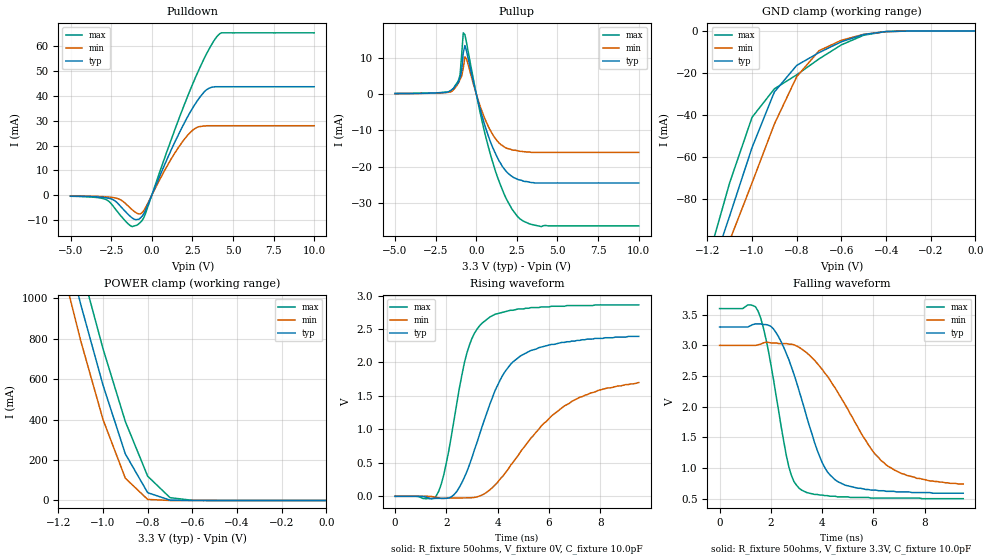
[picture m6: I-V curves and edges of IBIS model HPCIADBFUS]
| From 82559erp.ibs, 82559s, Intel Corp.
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[Model]   HPCIADBFUS
Model_type   I/O
Vinl  =   1.08V   | note : 0.3 * VCCmax
Vinh  =   1.5V   | note : 0.5 * VCCmin
|   typ   min  max
C_comp   2.7pF NA   NA
| note : on die power/gnd supply distribution R/L/C
|   are not included in the simulation
| note : pull up  mos are not active  pup#="1"
| note : POWER_clamp ref = VIO = VREF = 5.0V
|variable   typ   min   max
[Voltage range]   3.3V   3.0V   3.6V
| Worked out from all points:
|   slope of the pulldown table from 0 to 0.495 V, typ, clamps not added: 63.8 ohm
|   slope of the pullup table from 0 to 0.495 V, typ, clamps not added: 60.6 ohm
|   GND clamp passes 1 mA (typ) near -0.45 V on its own axis
|   POWER clamp passes 1 mA (typ) near -0.66 V on its own axis
|   rising waveform, R_fixture 50ohms, V_fixture 0V, C_fixture 10.0pF: 20-80 % time 1.48ns typ, 2.37ns min, 890ps max; typ from 0 V to 2.39 V
|   falling waveform, R_fixture 50ohms, V_fixture 3.3V, C_fixture 10.0pF: 20-80 % time 1.25ns typ, 2.04ns min, 777ps max; typ from 3.3 V to 0.59 V
| note : all DC curves are with 0.2 OHM res. in series to the PAD.
[GND_clamp]
|Voltage   I(typ)   I(min)   I(max)
-5V       -1.63A     -1.47A     -1.85A
-1.2V     -120mA     -130mA     -110mA
-1.1V     -88.2mA    -100mA     -72.4mA
-1V       -55.6mA    -72.5mA    -41.2mA
-900mV    -29.1mA    -44.4mA    -27.6mA
-800mV    -16.4mA    -21.8mA    -20.9mA
-700mV    -10.3mA    -9.39mA    -13.3mA
-600mV    -5.12mA    -4.42mA    -6.6mA
-500mV    -1.67mA    -1.57mA    -2mA
-400mV    -240uA     -300uA     -220uA
0V        0A         0A         0A
[PullDown]
|Voltage   I(typ)   I(min)   I(max)
-5V       -320uA     -230uA     -400uA
-2.8V     -1.01mA    -630uA     -1.76mA
-2.2V     -2.55mA    -1.14mA    -5.85mA
-1.4V     -8.01mA    -4.64mA    -11.8mA
-900mV    -9.77mA    -7.25mA    -12mA
-400mV    -6.32mA    -5.21mA    -7.64mA
1.2V      18.3mA     14.7mA     22.4mA
2.2V      31.5mA     24.1mA     39.7mA
3.3V      42.1mA     27.9mA     56mA
4V        43.7mA     28mA       63.8mA
4.3V      43.7mA     28mA       65.4mA
10V       43.7mA     28mA       65.4mA
[POWER_clamp]
|Voltage  I(typ)   I(min)   I(max)
-5V       20A        19.9A      20.2A
-1.2V     1.41A      1.23A      1.6A
-1.1V     970mA      790mA      1.16A
-1V       570mA      400mA      750mA
-900mV    230mA      110mA      390mA
-800mV    38.5mA     5.23mA     120mA
-700mV    1.75mA     120uA      14mA
-600mV    72.2uA     5.85uA     820uA
0V        1.93uA     1.69uA     2.17uA
[PullUp]
|Voltage  I(typ)   I(min)   I(max)
-5V       97.3uA     74.4uA     100uA
-1.4V     1.53mA     1.16mA     1.52mA
-1V       4.52mA     3.93mA     5.14mA
-800mV    11.3mA     7.1mA      16.8mA
-700mV    13.3mA     10.2mA     16.3mA
-600mV    11.8mA     9.65mA     14.1mA
300mV     -5.18mA    -4.13mA    -6.38mA
1.1V      -15.6mA    -11.8mA    -20.1mA
1.8V      -21.1mA    -14.8mA    -28.4mA
2.6V      -23.6mA    -15.7mA    -34mA
4V        -24.5mA    -16.1mA    -36.5mA
10V       -24.5mA    -16.1mA    -36.3mA
[Ramp]
| note : pad parasitics are not included
|Variable   typ   min   max
dV/dt_r   1.43/1.25n   1.03/2.1n   1.72/1.2n
dV/dt_f   1.63/1.2n   1.36/2.0n   1.86/0.7n
R_load =   50ohms
[Rising Waveform]
| note : pad parasitics are not included
| note : input changes at T=0.5nS
R_fixture   = 50ohms
V_fixture   = 0V
C_fixture   = 10.0pF
|Time   typ(V)   min(V)   max(V)
0s        32.32nV    49.99nV    20.75nV
1.7ns     -30.25mV   -22.52mV   72.53mV
1.9ns     -30.93mV   -30.7mV    320mV
2.3ns     24.49mV    -24.77mV   1.14V
2.8ns     370mV      -23.06mV   2.14V
3.4ns     1.05V      20.81mV    2.59V
4.1ns     1.74V      260mV      2.74V
4.9ns     2.1V       670mV      2.8V
6.9ns     2.32V      1.42V      2.85V
9.5ns     2.39V      1.7V       2.86V
[Falling Waveform]
| note : pad parasitics are not included
| note : input changes at T=0.5nS
R_fixture   = 50ohms
V_fixture   = 3.3V
V_fixture_min   = 3.0V
V_fixture_max   = 3.6V
C_fixture   = 10.0pF
|Time   typ   min   max
0s        3.3V       3V         3.6V
1.5ns     3.35V      3.01V      3.56V
1.8ns     3.34V      3.05V      3.12V
2.1ns     3.27V      3.04V      2.45V
2.7ns     2.77V      3.02V      1.02V
3.1ns     2.26V      2.97V      670mV
4ns       1.09V      2.61V      560mV
4.6ns     780mV      2.24V      530mV
6.5ns     620mV      1.05V      510mV
9.5ns     590mV      740mV      500mV
